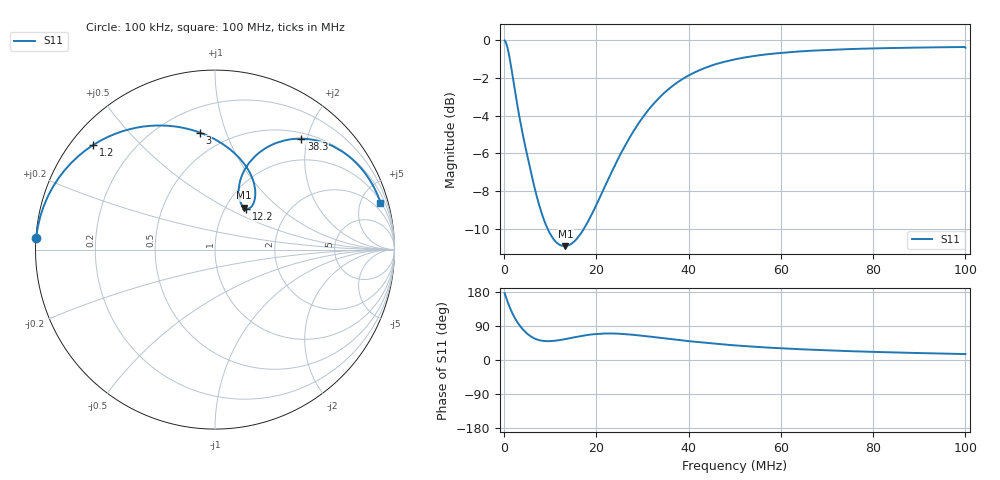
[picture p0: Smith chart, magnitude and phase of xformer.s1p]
# Hz S RI R 50.0
! written by SimSmith version 18.3h
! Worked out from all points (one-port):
!   1000 points, 100 kHz to 100 MHz, reference 50 ohm
!   lowest |S11| = -10.9 dB at 13.3 MHz (marker M1), VSWR 1.79, Z = 60.7 + j30.9 ohm
!   |S11| at or under -10 dB: 9.41 MHz to 17.31 MHz (7.897 MHz wide, 59.1 % of centre)
!   S11 on the Smith chart (normalised r, x): 100 kHz: 0.00, +0.03; 1.2 MHz: 0.06, +0.37; 3 MHz: 0.36, +0.82; 12.2 MHz: 1.25, +0.62; 38.3 MHz: 0.59, +1.90; 100 MHz: 1.21, +7.08
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100000  -0.9963 0.0636
600000  -0.9018 0.3517
900000  -0.7991 0.4849
1200000  -0.6795 0.5821
1600000  -0.5163 0.6592
2000000  -0.3657 0.6893
2500000  -0.2074 0.6839
3000000  -0.0835 0.6519
3600000  0.027 0.5983
4300000  0.1161 0.53
5800000  0.2091 0.3947
7100000  0.2245 0.3116
8500000  0.2152 0.2595
1.22e7  0.1726 0.228
1.26e7  0.1686 0.2296
1.33e7  0.162 0.2335
1.62e7  0.1406 0.2672
1.97e7  0.1322 0.3343
2.51e7  0.1758 0.4628
3.14e7  0.3076 0.5794
3.76e7  0.4647 0.6182
3.83e7  0.4813 0.6182
4.41e7  0.6033 0.5975
5.01e7  0.696 0.5543
6.26e7  0.8117 0.4557
7.51e7  0.8702 0.3743
8.76e7  0.9029 0.311
1e8  0.9197 0.2574
